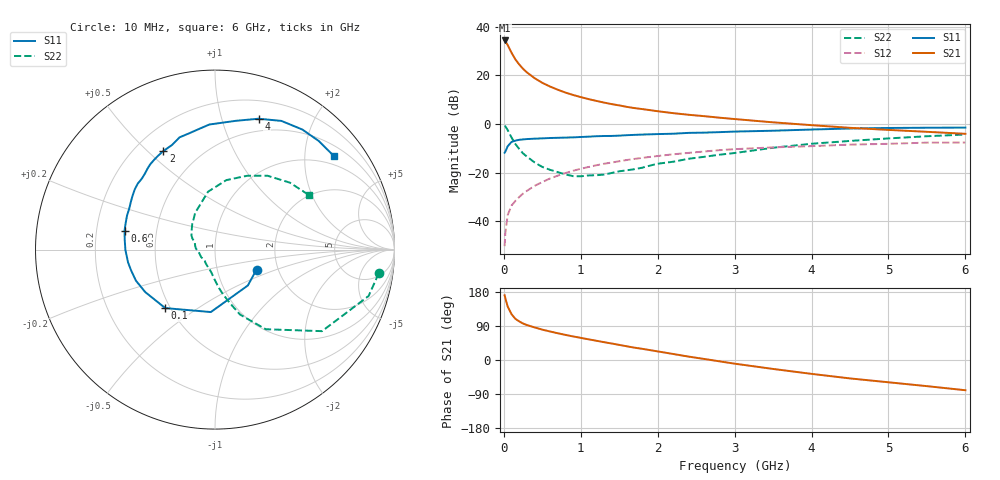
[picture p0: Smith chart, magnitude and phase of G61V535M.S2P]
! SIEMENS Small Signal Semiconductors
! BFG193
! Si NPN RF Bipolar Junction Transistor in SOT223
! VCE = 1.5 V  IC = 35 mA
! Common Emitter S-Parameters:  August  1996
# GHz  S  MA  R  50
!  f  S11  S21  S12  S22
! GHz  MAG  ANG  MAG  ANG  MAG  ANG  MAG  ANG
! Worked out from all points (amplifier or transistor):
!   36 points, 10 MHz to 6 GHz, reference 50 ohm
!   highest |S21| = 34.3 dB at 10 MHz (marker M1)
!   |S21| within 3 dB of that: start of sweep to 67.79 MHz
!   unconditionally stable (mu >= 1): 457.1 MHz to 2.683 GHz
!   at 250 MHz: K = 0.88, MSG = 25.6 dB, |S12| = -28.6 dB
!   at 1.4 GHz: K = 1.06, MAG = 10.5 dB, |S12| = -15.8 dB
!   at 6 GHz: K = 0.94, MSG = 1.8 dB, |S12| = -7.6 dB
!   S11 on the Smith chart (normalised r, x): 10 MHz: 1.55, -0.37; 100 MHz: 0.47, -0.38; 600 MHz: 0.32, +0.09; 2 GHz: 0.31, +0.56; 4 GHz: 0.37, +1.32; 6 GHz: 0.75, +2.70
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0.01  0.2567 -25.6  51.77 170.7  0.0031 87.6  0.9217 -8.3
0.02  0.2711 -47.5  49.84 162.7  0.0059 78.1  0.8941 -16.8
0.05  0.3487 -93.8  41.68 141.0  0.0135 68.3  0.7498 -37.3
0.1  0.428 -130.4  29.05 120.9  0.0212 62.5  0.5261 -57.5
0.15  0.4551 -148.7  21.16 108.6  0.0263 60.0  0.3884 -68.9
0.2  0.4732 -158.5  16.64 101.8  0.0317 61.3  0.3067 -74.7
0.25  0.4817 -166.1  13.54 96.3  0.0373 62.7  0.2481 -80.3
0.3  0.4896 -171.6  11.44 92.2  0.0424 64.2  0.2138 -84.3
0.4  0.4991 -179.7  8.702 86.0  0.0537 64.5  0.1621 -91.7
0.5  0.506 173.8  6.987 80.1  0.0641 63.8  0.1311 -98.3
0.6  0.5149 168.1  5.867 75.3  0.076 63.2  0.1146 -105.3
0.8  0.5254 158.9  4.412 66.3  0.0981 60.4  0.0923 -123.7
1.1  0.5486 146.9  3.24 54.6  0.1307 55.2  0.0878 -151.4
1.6  0.5881 129.6  2.241 36.1  0.1822 43.9  0.112 169.7
2  0.6198 117.7  1.825 22.7  0.2198 34.6  0.1528 149.0
2.2  0.6304 112.3  1.668 15.9  0.2383 29.8  0.1676 140.9
2.8  0.6792 97.2  1.347 -3.4  0.2895 15.4  0.2336 118.3
3.5  0.7265 80.9  1.08 -23.6  0.3306 -2.2  0.3248 96.9
4  0.7685 71.6  0.945 -36.6  0.3504 -12.0  0.3925 80.7
4.5  0.8069 62.7  0.833 -48.6  0.3768 -21.9  0.4485 66.5
5.5  0.8369 46.3  0.69 -69.0  0.4139 -44.6  0.5596 41.8
6  0.8429 38.2  0.628 -79.8  0.4155 -57.6  0.6067 29.9
